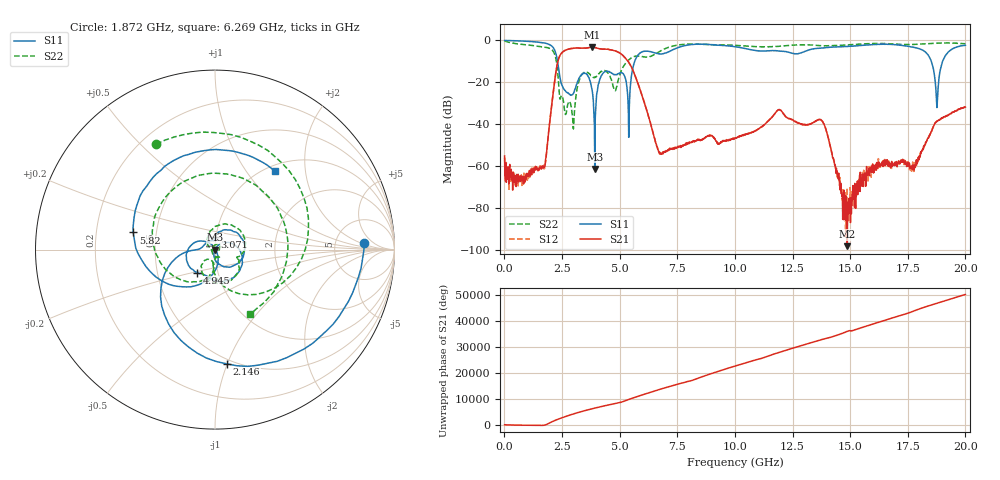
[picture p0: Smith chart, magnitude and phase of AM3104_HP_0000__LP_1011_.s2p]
!Created with skrf (http://scikit-rf.org).
# Hz S RI R 50.0
!freq ReS11 ImS11 ReS21 ImS21 ReS12 ImS12 ReS22 ImS22
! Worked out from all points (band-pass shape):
!   1601 points, 10 MHz to 20 GHz, reference 50 ohm
!   highest |S21| = -3.20 dB at 3.808 GHz (marker M1); lowest = -98.1 dB at 14.88 GHz (marker M2)
!   |S21| within 3 dB of the highest: 2.467 GHz to 5.041 GHz (2.574 GHz wide, 68.6 % of centre)
!   lowest |S11| = -61.3 dB at 3.921 GHz (marker M3), VSWR 1.00, Z = 50 - j0.0751 ohm
!   |S11| at or under -10 dB: 2.306 GHz to 5.651 GHz (3.345 GHz wide, 84.1 % of centre); 18.52 GHz to 19.01 GHz (486.2 MHz wide, 2.59 % of centre)
!   |S22| runs from -42.2 to -0.2 dB; largest |S21 - S12| = 0.007
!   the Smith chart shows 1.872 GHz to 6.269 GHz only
!   S11 on the Smith chart (normalised r, x): 1.872 GHz: 10, +3; 2.146 GHz: 0.46, -1.00; 3.071 GHz: 0.99, +0.14; 4.945 GHz: 0.80, -0.21; 5.82 GHz: 0.37, +0.09; 6.269 GHz: 1.11, +1.38
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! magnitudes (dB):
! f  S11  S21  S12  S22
! 10 MHz  0.0  -55.1  -55.9  -0.2
! 847.1 MHz  -0.3  -66.8  -63.3  -2.0
! 1.872 GHz  -1.6  -48.9  -49.2  -3.4
! 2.146 GHz  -3.9  -22.4  -22.4  -5.7
! 2.609 GHz  -23.6  -4.9  -4.9  -33.3
! 3.071 GHz  -23.1  -3.7  -3.6  -30.3
! 3.346 GHz  -16.2  -3.7  -3.7  -16.6
! 3.808 GHz  -23.7  -3.2  -3.2  -17.2
! 3.921 GHz  -61.3  -3.4  -3.4  -17.6
! 4.945 GHz  -15.8  -5.6  -5.6  -18.8
! 5.395 GHz  -46.2  -10.4  -10.4  -9.3
! 5.82 GHz  -6.6  -21.3  -21.3  -7.4
! 6.269 GHz  -5.2  -36.8  -36.8  -7.8
! 6.682 GHz  -6.3  -52.8  -52.7  -5.6
! 10.01 GHz  -2.9  -46.5  -46.6  -2.3
! 13.34 GHz  -4.1  -39.6  -39.5  -2.2
! 13.88 GHz  -3.5  -40.2  -40.3  -2.6
! 14.88 GHz  -2.9  -98.1  -77.7  -2.1
! 16.68 GHz  -1.8  -58.0  -58.0  -1.5
! 18.28 GHz  -5.6  -48.7  -48.5  -1.6
! 18.76 GHz  -32.0  -38.6  -38.5  -1.3
! 20 GHz  -2.3  -31.8  -31.7  -1.6
